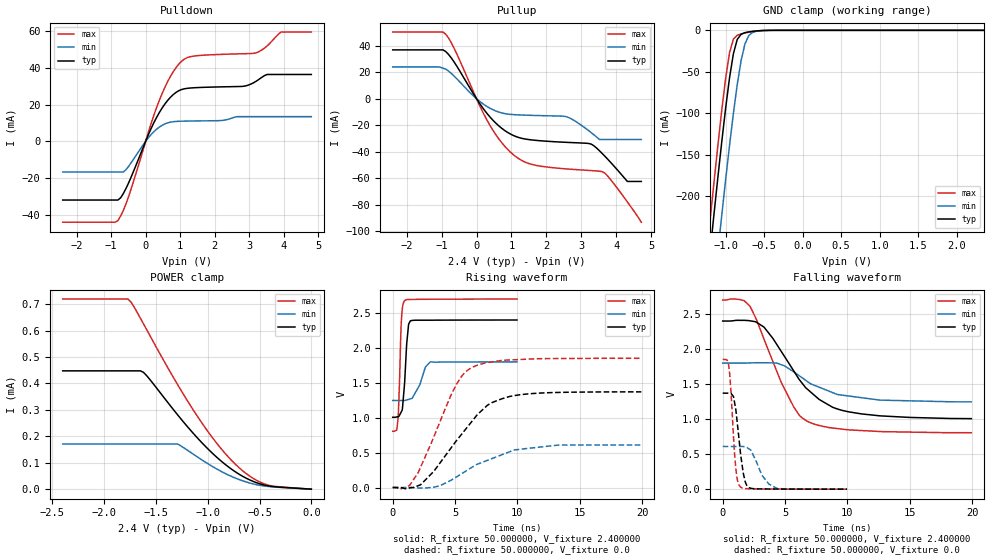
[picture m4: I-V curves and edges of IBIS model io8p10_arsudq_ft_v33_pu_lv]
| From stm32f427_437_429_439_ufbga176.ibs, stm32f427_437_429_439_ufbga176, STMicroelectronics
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|   Model io8p10_arsudq_ft_v33_pu_lv
[Model]  io8p10_arsudq_ft_v33_pu_lv
Model_type I/O
Polarity   Non-Inverting
Enable   Active-Low
Vinl =   0.720000V
Vinh =   1.680000V
Vmeas =  1.200000V
Cref =   40.000000pF
Rref =   100.000000M
Vref =   0.0V
C_comp   2.238700pF   2.180600pF   2.332300pF
[Temperature Range]   25.000000   0.125000k   -40.000000
[Pullup Reference]   2.400000V   1.800000V   2.700000V
[Pulldown Reference]   0.0V   0.0V   0.0V
[POWER Clamp Reference]   2.400000V   1.800000V   2.700000V
[GND Clamp Reference]   0.0V   0.0V   0.0V
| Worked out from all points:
|   slope of the pulldown table from 0 to 0.36 V, typ, clamps not added: 25 ohm
|   slope of the pullup table from 0 to 0.36 V, typ, clamps not added: 27.7 ohm
|   GND clamp passes 1 mA (typ) near -0.62 V on its own axis
|   rising waveform, R_fixture 50.000000, V_fixture 2.400000: 20-80 % time 302ps typ, 745ps min, 199ps max; typ from 1.01 V to 2.4 V
|   rising waveform, R_fixture 50.000000, V_fixture 0.0: 20-80 % time 3.63ns typ, 4.17ns min, 2.7ns max; typ from 0.001 V to 1.37 V
|   falling waveform, R_fixture 50.000000, V_fixture 2.400000: 20-80 % time 3.57ns typ, 3.54ns min, 2.74ns max; typ from 2.4 V to 1.01 V
|   falling waveform, R_fixture 50.000000, V_fixture 0.0: 20-80 % time 535ps typ, 1.04ns min, 388ps max; typ from 1.37 V to 0.001 V
[Pulldown]
|Voltage   I(typ)   I(min)   I(max)
-2.4V     -31.73mA   -16.51mA   -43.74mA
-800mV    -31.73mA   -16.51mA   -42.87mA
-480mV    -21.98mA   -13.17mA   -29.21mA
80mV      3.63mA     1.966mA    5.014mA
480mV     18.16mA    8.738mA    26.02mA
800mV     25.38mA    10.72mA    37.77mA
1.12V     28.53mA    11.02mA    44.6mA
2.8V      29.84mA    13.45mA    47.53mA
3.2V      32.59mA    13.45mA    48.03mA
3.52V     36.3mA     13.45mA    51.74mA
3.92V     36.3mA     13.45mA    59.27mA
4.8V      36.3mA     13.45mA    59.27mA
[Pullup]
|Voltage   I(typ)   I(min)   I(max)
-2.4V     36.81mA    24mA       50.22mA
-960mV    36.81mA    23.01mA    50.22mA
-640mV    27.63mA    17.02mA    37.96mA
320mV     -11.75mA   -6.207mA   -17.08mA
640mV     -20.52mA   -10.1mA    -30.35mA
960mV     -26.47mA   -11.82mA   -40.02mA
1.52V     -30.88mA   -12.51mA   -49.05mA
2.56V     -32.88mA   -13.48mA   -52.9mA
3.28V     -34.18mA   -25.5mA    -54.17mA
3.6V      -41.3mA    -30.74mA   -54.97mA
4.32V     -62.38mA   -30.74mA   -77.8mA
4.72V     -62.38mA   -30.74mA   -93.1mA
[GND_clamp]
|Voltage   I(typ)   I(min)   I(max)
-2.4V     -1.424A    -1.508A    -1.394A
-1.25V    -311.2mA   -401.9mA   -273.3mA
-1.2V     -265.4mA   -356.1mA   -227.2mA
-1.15V    -220.4mA   -310.8mA   -181.9mA
-1.1V     -176.3mA   -266.2mA   -137.9mA
-1.05V    -133.8mA   -222.5mA   -95.87mA
-950mV    -57.3mA    -138.9mA   -26.98mA
-900mV    -28.27mA   -100.4mA   -10.59mA
-850mV    -11.01mA   -65.54mA   -5.958mA
-750mV    -2.834mA   -16.5mA    -3.178mA
-600mV    -750uA     -1.164mA   -738.3uA
2.35V     0A         0A         0A
[POWER_clamp]
|Voltage   I(typ)   I(min)   I(max)
-2.4V     447.7uA    170.8uA    719.3uA
-1.77V    447.7uA    170.8uA    719.3uA
-1.74V    447.7uA    170.8uA    707.6uA
-1.65V    447.7uA    170.8uA    647uA
-1.62V    442uA      170.8uA    625.5uA
-1.29V    280.9uA    170.8uA    395.1uA
-1.02V    161uA      101.5uA    230.1uA
-780mV    78.34uA    49.93uA    112.9uA
-600mV    36.03uA    23.94uA    50.74uA
-450mV    15.19uA    11.76uA    19.45uA
-330mV    8.429uA    7.427uA    9.749uA
0V        0A         0A         0A
[Ramp]
| variable   typ   min   max
dV/dt_r  0.82207/3.62819n   0.36578/4.17472n   1.11311/2.70023n
dV/dt_f  0.83316/3.57481n   0.33360/3.58870n   1.13593/2.74274n
R_load = 50.000000
[Rising Waveform]
R_fixture= 50.000000
V_fixture= 2.400000
V_fixture_min= 1.800000
V_fixture_max= 2.700000
|time   V(typ)   V(min)   V(max)
0s        1.007V     1.247V     806mV
320.3ps   1.012V     1.247V     824.1mV
440.4ps   1.017V     1.247V     1.003V
680.7ps   1.082V     1.247V     2.336V
800.8ps   1.173V     1.247V     2.602V
961ps     1.516V     1.247V     2.676V
1.121ns   2.057V     1.255V     2.691V
1.421ns   2.388V     1.271V     2.694V
3.023ns   2.397V     1.801V     2.697V
9.97ns    2.4V       1.8V       2.7V
[Rising Waveform]
R_fixture= 50.000000
V_fixture= 0.0
V_fixture_min= 0.0
V_fixture_max= 0.0
|time   V(typ)   V(min)   V(max)
0s        954.9uV    874.9uV    1.146mV
1.361ns   -4.945mV   345.5uV    31.99mV
2.042ns   26.64mV    -5.38mV    214.7mV
3.283ns   230.6mV    5.237mV    719.6mV
4.805ns   598.3mV    118.2mV    1.373V
5.566ns   772.8mV    203mV      1.604V
6.366ns   951.1mV    292.3mV    1.72V
7.608ns   1.181V     390.8mV    1.791V
9.77ns    1.318V     540.1mV    1.831V
19.94ns   1.371V     610.3mV    1.852V
[Falling Waveform]
R_fixture= 50.000000
V_fixture= 2.400000
V_fixture_min= 1.800000
V_fixture_max= 2.700000
|time   V(typ)   V(min)   V(max)
0s        2.4V       1.8V       2.7V
1.602ns   2.41V      1.8V       2.696V
2.202ns   2.403V     1.802V     2.607V
3.323ns   2.311V     1.805V     2.137V
4.725ns   1.959V     1.775V     1.513V
6.086ns   1.579V     1.626V     1.07V
6.767ns   1.431V     1.54V      971.7mV
8.809ns   1.17V      1.379V     873.8mV
10.13ns   1.104V     1.33V      846.8mV
19.94ns   1.007V     1.247V     806mV
[Falling Waveform]
R_fixture= 50.000000
V_fixture= 0.0
V_fixture_min= 0.0
V_fixture_max= 0.0
|time   V(typ)   V(min)   V(max)
0s        1.371V     610.3mV    1.852V
460.5ps   1.371V     610.1mV    1.79V
660.7ps   1.367V     610mV      1.396V
1.041ns   1.145V     609.8mV    314.8mV
1.421ns   522.1mV    610.7mV    32.77mV
1.802ns   109.1mV    606.7mV    9.273mV
2.202ns   16.43mV    564.5mV    6.048mV
3.143ns   4.431mV    199.9mV    3.852mV
4.364ns   2.674mV    11.14mV    2.477mV
9.97ns    954.9uV    874.9uV    1.146mV
